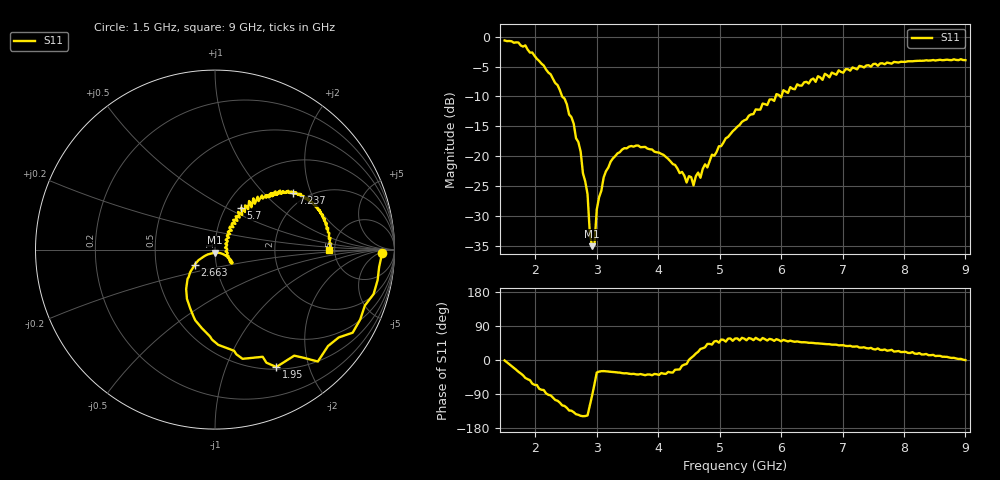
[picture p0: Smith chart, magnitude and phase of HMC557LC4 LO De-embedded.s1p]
! Hittite Microwave Corporation
! 20 Alpha Road
! Chelmsford, MA 01824
! http://www.hittite.com
! Tel: 978-250-3343
! Fax: 978-250-3373
! Device:  HMC557LC4
! Description: GaAS MMIC Fundamental  Mixer
! Frequency:  2.5 -  7.0 GHz
! Package:  LC4  - Ceramic- 24 pins
! Ports:  1,LO Port De-embedd from: 1.5GHz-9GHz @ 15dBm power
! Data:  The device was measured on evaluation board 118703.
!  The evaluation circuit board was modeled and simulated.  This was use
!  to removed the evaluation board circuit from the measured data.
!  The reference plane is the center of the package pin.
! Misc:
! Date Measured:  20-02-2008
! Date:  21-02-2008
! Note:
!  Hittite supplies this data as a sample of measured data at the package pin for
!  for this package product.  Your particular data for this product may vary.
!  Data was taken at 25 degrees C.
!  Hittite reserves the right to change this data at anytime# MHz S MA R 50
# MHz S MA R 50
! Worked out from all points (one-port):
!   201 points, 1.5 GHz to 9 GHz, reference 50 ohm
!   lowest |S11| = -35.1 dB at 2.925 GHz (marker M1), VSWR 1.04, Z = 49.9 - j1.75 ohm
!   |S11| at or under -10 dB: 2.437 GHz to 5.912 GHz (3.475 GHz wide, 83.3 % of centre); 5.986199 GHz to 6.004605 GHz (18.41 MHz wide, 0.307 % of centre)
!   S11 on the Smith chart (normalised r, x): 1.5 GHz: 26, -7; 1.95 GHz: 0.53, -1.52; 2.663 GHz: 0.79, -0.14; 5.7 GHz: 1.18, +0.60; 7.237 GHz: 1.70, +1.49; 9 GHz: 4.51, -0.06
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1500  0.9316 -1.1
1725  0.8959 -31.1
1837.5  0.8469 -47.4
1950  0.738 -62.4
2175  0.5309 -88.1
2437.5  0.3154 -119.8
2625  0.1869 -137.8
2662.5  0.1413 -143.1
2737.5  0.1093 -147.3
2775  0.07188 -148.3
2850  0.04798 -146.2
2887.5  0.02237 -119.7
2925  0.01761 -93.2
2962.5  0.01801 -63.9
3000  0.03573 -33.1
3112.5  0.06641 -29.4
3375  0.108 -33.3
3787.5  0.1196 -40.1
4312.5  0.07877 -25.2
4575  0.05688 10.8
4650  0.07281 21.7
5250  0.1683 56.6
5700  0.2758 58.1
6187.5  0.3666 49.2
7125  0.5204 37.4
7237.5  0.5336 36.0
8062.5  0.6233 18.8
9000  0.6369 -0.3
